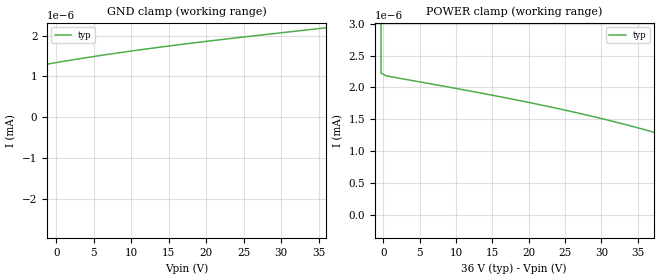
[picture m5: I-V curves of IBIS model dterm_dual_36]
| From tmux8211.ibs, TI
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| dterm_dual_36
[Model]   dterm_dual_36
Model_type   Terminator
|   typ   min   max
C_comp   4.014581e-12   NA   NA
[Voltage Range]   36   NA   NA
[Temperature Range]   27   NA   NA
[Power Clamp Reference]   36   NA   NA
[GND Clamp Reference]   0   NA   NA
[GND Clamp]
|   Voltage   I(typ)   I(min)   I(max)
-41V      -1.446A    NA         NA
-36.33V   -6.504nA   NA         NA
-35.56V   -237.3pA   NA         NA
-33.22V   -198.1pA   NA         NA
-30.89V   -118.5pA   NA         NA
-20V      499.9pA    NA         NA
-15.33V   741.1pA    NA         NA
-9.111V   1.014nA    NA         NA
-2.889V   1.243nA    NA         NA
4.111V    1.46nA     NA         NA
12.67V    1.686nA    NA         NA
36V       2.19nA     NA         NA
[POWER Clamp]
|   Voltage   I(typ)   I(min)   I(max)
-5V       744mA      NA         NA
-1.111V   26.13mA    NA         NA
-333.3mV  2.226nA    NA         NA
444.4mV   2.181nA    NA         NA
23.78V    1.675nA    NA         NA
32.33V    1.447nA    NA         NA
39.33V    1.227nA    NA         NA
45.56V    996.4pA    NA         NA
51.78V    719.6pA    NA         NA
66.56V    -103.6pA   NA         NA
68.89V    -189.6pA   NA         NA
72V       -243pA     NA         NA
